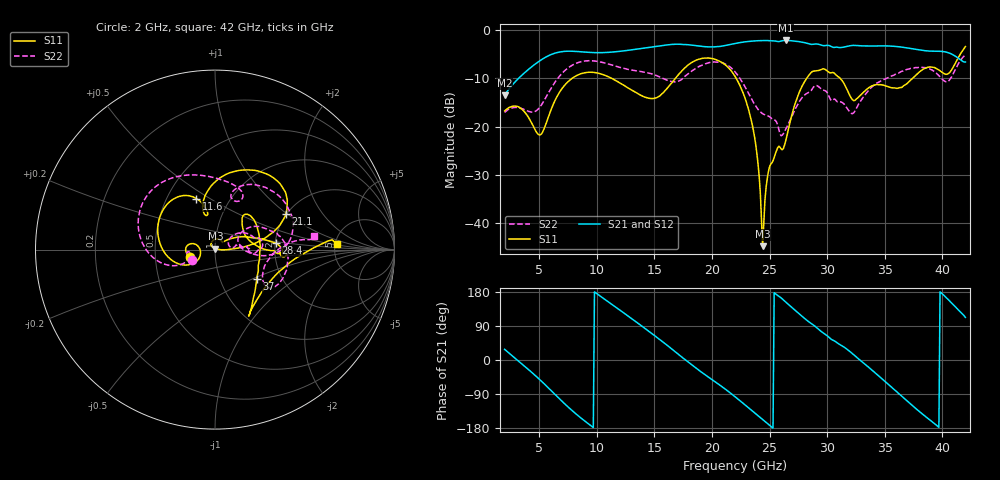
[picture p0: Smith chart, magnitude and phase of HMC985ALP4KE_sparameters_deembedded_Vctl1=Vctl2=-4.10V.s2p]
!s2p File: Measurements: S11, S21, S12, S22
# GHz S dB R 50.0
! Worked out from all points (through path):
!   401 points, 2 GHz to 42 GHz, reference 50 ohm
!   highest |S21| = -2.09 dB at 26.4 GHz (marker M1); lowest = -13.5 dB at 2 GHz (marker M2)
!   lowest |S11| = -44.9 dB at 24.4 GHz (marker M3), VSWR 1.01, Z = 50.2 + j0.54 ohm
!   |S11| at or under -10 dB: start of sweep to 7.843 GHz; 22.11 GHz to 28.21 GHz (6.104 GHz wide, 24.3 % of centre); 31.14 GHz to 37.4 GHz (6.254 GHz wide, 18.3 % of centre)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
!   |S22| runs from -21.9 to -5.1 dB; largest |S21 - S12| = 0.00061
!   S11 on the Smith chart (normalised r, x): 2 GHz: 0.75, -0.07; 11.6 GHz: 0.70, +0.44; 21.1 GHz: 1.98, +0.99; 28.4 GHz: 2.01, +0.16; 37 GHz: 1.49, -0.53; 42 GHz: 5.14, +0.61
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2  -16.74 -162.4  -13.47 28.1  -13.48 28.2  -17.07 -156.3
5.1  -21.71 -169.4  -6.25 -53.1  -6.25 -53.1  -15.82 -159.5
6.3  -14.95 -151.3  -4.79 -88.6  -4.79 -88.6  -11.03 -162.3
8.7  -8.96 149.8  -4.46 -154.9  -4.46 -154.9  -6.47 150.8
11.6  -10.37 110.1  -4.46 140.5  -4.46 140.5  -7.41 103.0
13.6  -13.21 101.6  -3.85 96.5  -3.85 96.5  -8.47 75.2
15.4  -13.73 106.7  -3.25 55.5  -3.25 55.6  -9.61 62.1
17.9  -7.25 79.4  -2.97 -4.7  -2.98 -4.7  -9.09 71.9
21.1  -7.07 26.9  -3.17 -75.5  -3.17 -75.5  -6.94 15.2
22  -9.53 16.5  -2.73 -96.8  -2.73 -96.8  -8.61 -0.1
23.5  -19.63 2.6  -2.23 -134.2  -2.23 -134.2  -14.53 -4.7
24.4  -44.86 70.1  -2.12 -156.9  -2.12 -156.8  -17.33 8.5
25  -28.32 127.1  -2.14 -172.2  -2.14 -172.2  -17.95 12.1
26.4  -22.98 41.6  -2.09 153.0  -2.09 153.1  -20.55 33.8
28.4  -9.37 5.9  -2.77 100.9  -2.78 100.9  -12.90 17.4
28.7  -8.57 0.9  -2.91 94.8  -2.91 94.8  -12.18 15.6
32.4  -14.56 30.4  -3.12 11.3  -3.12 11.3  -16.82 26.7
33.9  -11.52 47.9  -3.25 -26.9  -3.25 -26.8  -11.72 30.1
35.4  -11.75 17.5  -3.25 -66.9  -3.25 -66.8  -9.72 18.6
37  -10.90 -35.2  -3.67 -110.0  -3.67 -110.0  -8.08 3.9
39.8  -8.41 -56.0  -4.35 179.8  -4.35 179.8  -9.65 -34.4
42  -3.37 2.7  -6.57 112.3  -6.57 112.3  -5.12 7.6
